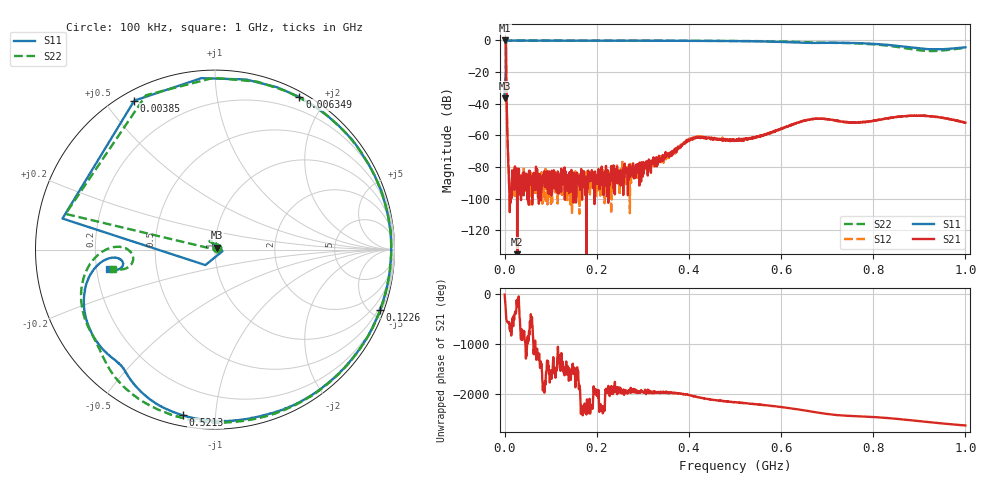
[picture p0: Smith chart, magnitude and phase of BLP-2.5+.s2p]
! Mini-Circuits
! S2P DATA File Format
! Type: LOW PASS FILTER
! Model:BLP-2.5+
! All S Parameters are in dB deg format
! TEST CONDITIONS: INPUT POWER = 0 dBm @ Temperature = +25 deg C
! 1601 Frequency points
# MHz S DB R 50
!FREQMAG(S11)PHS(S11)MAG(S21)PHS(S21)MAG(S12)PHS(S12)MAG(S22)PHS(S22)
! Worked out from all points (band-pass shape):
!   1601 points, 100 kHz to 1 GHz, reference 50 ohm
!   highest |S21| = -0.09 dB at 100 kHz (marker M1); lowest = -186.0 dB at 27.6 MHz (marker M2)
!   |S21| within 3 dB of the highest: start of sweep to 2.732 MHz
!   lowest |S11| = -36.6 dB at 100 kHz (marker M3), VSWR 1.03, Z = 51 + j1.14 ohm
!   |S11| at or under -10 dB: start of sweep to 2.931 MHz
!   |S22| runs from -36.5 to -0.1 dB; largest |S21 - S12| = 0.028
!   S11 on the Smith chart (normalised r, x): 100 kHz: 1.02, +0.02; 3.85 MHz: 0.04, +0.59; 6.349 MHz: 0.06, +1.70; 122.6 MHz: 0.35, -5.66; 521.3 MHz: 0.05, -0.82; 1 GHz: 0.25, -0.09
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0.1  -36.56 48.8  -0.09 -10.6  -0.08 -10.7  -36.53 48.3
1.974813  -27.42 -12.1  -0.54 134.8  -0.54 133.5  -26.41 95.3
3.849625  -0.50 118.5  -26.26 -145.9  -26.61 -146.7  -0.52 114.1
6.349375  -0.25 61.0  -61.79 155.6  -62.07 156.4  -0.26 57.8
8.224188  -0.22 45.2  -79.57 143.2  -77.91 133.5  -0.21 42.7
9.474062  -0.18 38.4  -89.47 163.8  -85.91 122.6  -0.20 36.3
11.97381  -0.18 29.3  -95.56 112.0  -101.57 161.3  -0.18 27.5
18.22319  -0.17 17.1  -86.42 140.8  -96.66 9.5  -0.16 15.9
27.59725  -0.16 8.3  -186.02 111.7  -89.70 -95.0  -0.15 7.4
58.84412  -0.18 -4.8  -87.18 141.9  -86.26 -108.0  -0.17 -5.5
122.5878  -0.18 -20.0  -95.72 132.6  -90.50 -94.0  -0.16 -20.9
166.9583  -0.19 -29.1  -85.60 -118.7  -87.74 -76.6  -0.17 -30.2
285.0715  -0.22 -52.6  -81.15 -132.1  -81.39 -172.1  -0.21 -54.3
333.8166  -0.26 -62.3  -75.70 -166.6  -75.97 -159.9  -0.23 -64.2
408.1842  -0.34 -77.1  -62.52 117.7  -62.19 124.4  -0.29 -79.5
500.6749  -0.46 -96.6  -63.01 -0.6  -62.83 -5.8  -0.38 -99.3
521.2979  -0.53 -101.1  -62.60 -19.6  -62.69 -19.6  -0.42 -103.8
666.9083  -1.61 -129.8  -49.73 170.7  -49.76 169.8  -1.31 -136.9
765.6484  -1.76 -151.3  -51.88 77.3  -51.90 76.7  -1.94 -158.7
833.7667  -2.92 -168.0  -49.10 39.9  -49.11 39.5  -3.48 -176.1
921.2579  -5.60 -173.5  -47.87 -39.8  -47.90 -39.6  -6.75 -175.7
1000  -4.40 -169.6  -52.03 -106.4  -51.88 -106.2  -4.73 -169.5
